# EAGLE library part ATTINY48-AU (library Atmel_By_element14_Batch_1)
8-bit Microcontroller
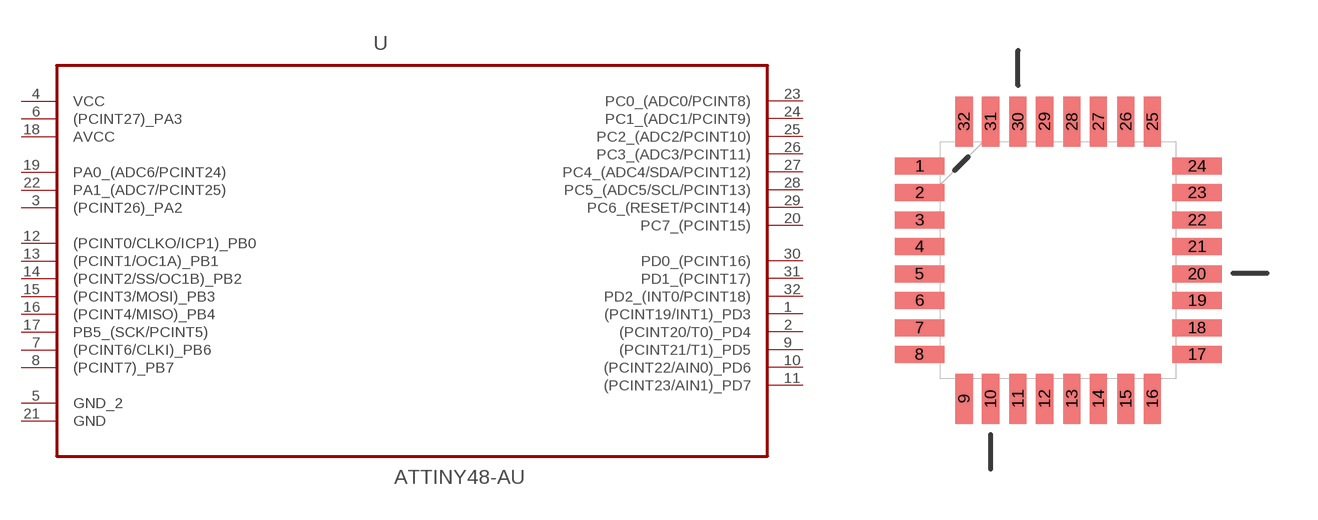
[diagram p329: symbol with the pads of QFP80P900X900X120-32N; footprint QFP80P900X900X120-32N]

Designator prefix U

## ATTINY48-AU (MPN: ATTINY48-AU; OC_FARNELL: 1636953; OC_NEWARK: 68T3768; PACKAGE: QFP-32; SUPPLIER: Atmel)  [QFP80P900X900X120-32N]
1  (PCINT19/INT1)_PD3
2  (PCINT20/T0)_PD4
3  (PCINT26)_PA2
4  VCC  pwr
5  GND_2  pas
6  (PCINT27)_PA3
7  (PCINT6/CLKI)_PB6
8  (PCINT7)_PB7
9  (PCINT21/T1)_PD5
10  (PCINT22/AIN0)_PD6
11  (PCINT23/AIN1)_PD7
12  (PCINT0/CLKO/ICP1)_PB0
13  (PCINT1/OC1A)_PB1
14  (PCINT2/SS/OC1B)_PB2
15  (PCINT3/MOSI)_PB3
16  (PCINT4/MISO)_PB4
17  PB5_(SCK/PCINT5)
18  AVCC  pwr
19  PA0_(ADC6/PCINT24)
20  PC7_(PCINT15)
21  GND  pas
22  PA1_(ADC7/PCINT25)
23  PC0_(ADC0/PCINT8)
24  PC1_(ADC1/PCINT9)
25  PC2_(ADC2/PCINT10)
26  PC3_(ADC3/PCINT11)
27  PC4_(ADC4/SDA/PCINT12)
28  PC5_(ADC5/SCL/PCINT13)
29  PC6_(RESET/PCINT14)
30  PD0_(PCINT16)
31  PD1_(PCINT17)
32  PD2_(INT0/PCINT18)

## Footprint QFP80P900X900X120-32N (pad centres in mm)
smd 1.473 x 0.508: 1 -4.115,2.794; 2 -4.115,2.007; 3 -4.115,1.194; 4 -4.115,0.406; 5 -4.115,-0.406; 6 -4.115,-1.194; 7 -4.115,-2.007; 8 -4.115,-2.794; 17 4.115,-2.794; 18 4.115,-2.007; 19 4.115,-1.194; 20 4.115,-0.406; 21 4.115,0.406; 22 4.115,1.194; 23 4.115,2.007; 24 4.115,2.794
smd 0.508 x 1.473: 9 -2.794,-4.115; 10 -2.007,-4.115; 11 -1.194,-4.115; 12 -0.406,-4.115; 13 0.406,-4.115; 14 1.194,-4.115; 15 2.007,-4.115; 16 2.794,-4.115; 25 2.794,4.115; 26 2.007,4.115; 27 1.194,4.115; 28 0.406,4.115; 29 -0.406,4.115; 30 -1.194,4.115; 31 -2.007,4.115; 32 -2.794,4.115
